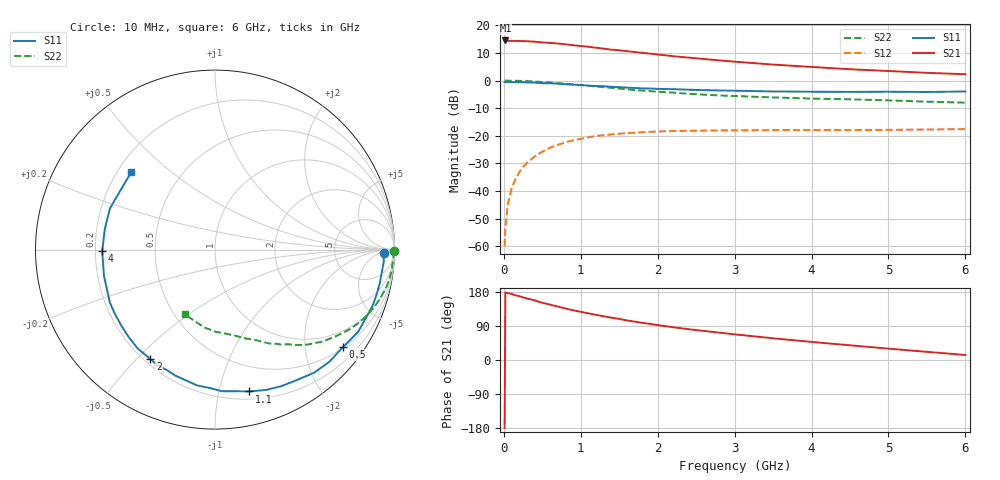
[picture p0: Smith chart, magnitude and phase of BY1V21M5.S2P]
! SIEMENS Small Signal Semiconductors
! BFY420
! Si NPN RF SIEGET Grounded Emitter Transistor in MICRO-X
! VCE = 1.25 V  IC = 1.5 mA
! Common Emitter S-Parameters:  October  1996
# GHz  S  MA  R  50
!  f  S11  S21  S12  S22
! GHz  MAG  ANG  MAG  ANG  MAG  ANG  MAG  ANG
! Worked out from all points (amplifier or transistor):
!   36 points, 10 MHz to 6 GHz, reference 50 ohm
!   highest |S21| = 14.5 dB at 20 MHz (marker M1)
!   |S21| within 3 dB of that: start of sweep to 1.307 GHz
!   unconditionally stable (mu >= 1): 4.245 GHz to end of sweep
!   at 250 MHz: K = 0.04, MSG = 22.8 dB, |S12| = -31.4 dB
!   at 1.4 GHz: K = 0.27, MSG = 15.4 dB, |S12| = -19.5 dB
!   at 6 GHz: K = 1.29, MAG = 6.7 dB, |S12| = -17.6 dB
!   S11 on the Smith chart (normalised r, x): 10 MHz: 31, -9; 500 MHz: 0.52, -2.88; 1.1 GHz: 0.27, -1.24; 2 GHz: 0.22, -0.55; 4 GHz: 0.23, -0.01; 6 GHz: 0.26, +0.37
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0.01  0.942 -1.0  5.317 -179.5  0.001 99.2  0.9984 -0.5
0.02  0.9385 -1.6  5.336 178.5  0.0021 89.4  0.9995 -0.8
0.05  0.9427 -4.0  5.255 176.5  0.0055 89.1  0.9956 -2.0
0.1  0.938 -7.8  5.235 174.6  0.011 84.1  0.992 -4.1
0.15  0.9372 -11.3  5.233 170.5  0.0163 82.7  0.9916 -6.2
0.2  0.9344 -15.2  5.209 168.5  0.0218 82.1  0.9884 -8.0
0.3  0.9264 -22.5  5.169 162.3  0.0322 76.8  0.978 -12.1
0.4  0.9197 -30.0  5.065 157.4  0.0421 72.2  0.9625 -16.0
0.5  0.8957 -37.3  4.916 150.9  0.0516 67.7  0.9439 -19.7
0.7  0.8803 -51.2  4.705 141.2  0.0686 59.6  0.9008 -26.8
0.8  0.8579 -57.9  4.544 136.0  0.0761 55.3  0.877 -30.0
1.1  0.8129 -76.4  4.108 123.1  0.094 45.7  0.8039 -38.5
1.4  0.7713 -92.3  3.634 111.7  0.1059 37.2  0.7396 -45.7
1.6  0.7445 -103.2  3.407 104.4  0.1122 32.4  0.6959 -49.8
2  0.7084 -120.5  2.97 92.0  0.1196 24.6  0.6286 -56.6
2.2  0.6989 -128.2  2.773 86.5  0.1219 21.4  0.6047 -59.9
2.8  0.6625 -147.5  2.324 72.2  0.1251 14.2  0.5384 -68.0
3.5  0.6355 -166.8  1.951 57.3  0.1269 8.7  0.4951 -76.3
4  0.6285 -179.2  1.767 47.7  0.1271 5.8  0.4723 -82.6
4.5  0.6246 169.5  1.605 38.8  0.1272 3.4  0.4577 -89.4
5.5  0.6216 147.5  1.383 21.5  0.1298 1.2  0.4148 -105.5
6  0.6356 137.2  1.304 13.3  0.1322 0.8  0.3978 -114.9
